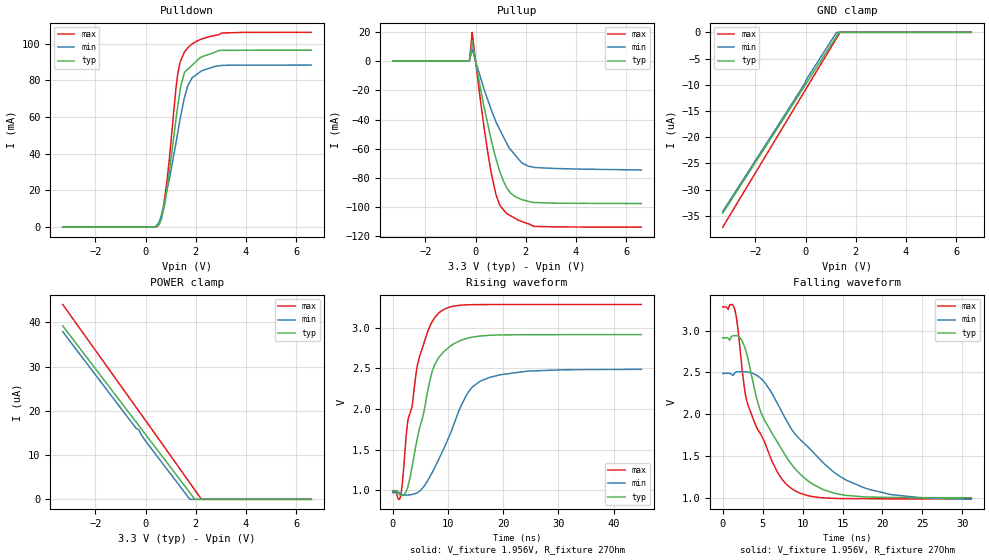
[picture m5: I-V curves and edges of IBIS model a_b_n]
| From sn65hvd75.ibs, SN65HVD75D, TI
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[Model]   a_b_n
Model_type   I/O
Polarity   Non-Inverting
Enable   Active-High
Vinl = 0.8
Vinh = 2.0
Vmeas = 1.65
Vref = 1.65
Cref = 50pF
Rref = 27
|   typ   min   max
|   (nom PVT)   (fast PVT)   (slow PVT)
C_comp   2.134e-11   2.058e-11   2.134e-11
|ON state : BUFFER OUTPUT TURNED HIGH
|C_comp   2.134e-11   2.058e-11   2.134e-11
|OFF state: BUFFER IN HIGH IMPEDANCE
|C_comp   1.142e-11   1.069e-11   1.206e-11
| Where nom  PVT is Nominal Process, 3.3V, 27C
|   Fast PVT is Strong Process,  3.6V, -40C
|   Slow PVT is Weak Process,   3V, 125C
[Voltage Range]   3.3   3   3.6
|Ambient Temperature   25   125   -40
|Junction Temperature
[Temperature Range]   27   125   -40
[Pullup Reference]   3.3   3   3.6
[Pulldown Reference]   0   0   0
[Power Clamp Reference]   3.3   3   3.6
[GND Clamp Reference]   0   0   0
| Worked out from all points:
|   slope of the pulldown table from 0 to 0.495 V, typ, clamps not added: 482 ohm
|   slope of the pullup table from 0 to 0.495 V, typ, clamps not added: 11.3 ohm
|   falling waveform, V_fixture 1.956V, R_fixture 27Ohm: 20-80 % time 5.29ns typ, 7.74ns min, 4.01ns max; typ from 2.92 V to 0.998 V
|   rising waveform, V_fixture 1.956V, R_fixture 27Ohm: 20-80 % time 3.78ns typ, 5.92ns min, 3.54ns max; typ from 0.997 V to 2.91 V
[Pulldown]
|   Voltage   I(typ)   I(min)   I(max)
-3.3V     0A         0A         0A
478.8mV   881.8uA    1.608mA    490.4uA
633.6mV   4.473mA    6.787mA    5.518mA
849.6mV   20.36mA    20.02mA    24.85mA
1.202V    57.94mA    45.29mA    74.75mA
1.285V    66.34mA    51.87mA    83.81mA
1.399V    76.97mA    60.61mA    90.81mA
1.554V    84.49mA    70.97mA    95.7mA
1.854V    88.36mA    81.44mA    99.95mA
2.168V    92.42mA    84.62mA    102.3mA
2.934V    96.41mA    88.05mA    105.1mA
6.6V      96.53mA    88.41mA    106.3mA
[GND Clamp]
|   Voltage   I(typ)   I(min)   I(max)
-3.3V     -34.49uA   -34.15uA   -37.14uA
-162mV    -11.16uA   -10.73uA   -12.21uA
111mV     -9.118uA   -8.406uA   -10.04uA
1.236V    -746.4nA   -6.684nA   -1.095uA
1.333V    -22.23nA   0A         -321.6nA
1.372V    0A         0A         -15.83nA
6.6V      0A         0A         0A
[Pullup]
|   Voltage   I(typ)   I(min)   I(max)
-3.3V     0A         0A         0A
-248.4mV  0A         0A         0A
-133.2mV  13.34mA    8.273mA    19.82mA
64.8mV    -6.244mA   -3.735mA   -9.275mA
342mV     -31.73mA   -19.41mA   -45.91mA
633.6mV   -54.97mA   -33.82mA   -77.49mA
802.8mV   -66.31mA   -41.19mA   -90.85mA
939.6mV   -74.34mA   -46.13mA   -97.84mA
1.213V    -85.9mA    -55.41mA   -104.1mA
1.554V    -92.65mA   -63.94mA   -107.6mA
2.115V    -96.23mA   -72.14mA   -111.7mA
6.6V      -97.64mA   -74.6mA    -113.8mA
[POWER Clamp]
|   Voltage   I(typ)   I(min)   I(max)
-3.3V     39.2uA     37.89uA    44.02uA
-378mV    17.47uA    16.05uA    20.8uA
-264mV    16.62uA    15.69uA    19.89uA
-150mV    15.78uA    14.44uA    18.99uA
6mV       14.61uA    13.14uA    17.75uA
1.761V    1.513uA    15.72nA    3.718uA
1.964V    2.365nA    0A         2.098uA
2.225V    0A         0A         12.85nA
6.6V      0A         0A         0A
[Ramp]
R_load = 27
|   typ   min   max
dV/dt_r   1.32254/4.33263e-09   0.977856/7.13635e-09   1.58731/3.88744e-09
dV/dt_f   1.15015/5.29718e-09   0.908154/7.76592e-09   1.38004/4.01751e-09
[Falling Waveform]
V_fixture = 1.956V
V_fixture_min = 1.731V
V_fixture_max = 2.134V
R_fixture = 27Ohm
C_fixture = 0F
|   Time   V(typ)   V(min)   V(max)
0s        2.915V     2.488V     3.285V
1.5ns     2.94V      2.492V     3.258V
2.44ns    2.876V     2.509V     2.531V
3.05ns    2.707V     2.506V     2.148V
4.79ns    2.02V      2.427V     1.753V
6.95ns    1.65V      2.11V      1.288V
8.58ns    1.402V     1.823V     1.11V
12.39ns   1.104V     1.435V     997.9mV
17.6ns    1.009V     1.121V     986mV
31.12ns   998.1mV    978.9mV    984.8mV
[Rising Waveform]
V_fixture = 1.956V
V_fixture_min = 1.731V
V_fixture_max = 2.134V
R_fixture = 27Ohm
C_fixture = 0F
|   Time   V(typ)   V(min)   V(max)
0s        996.9mV    973.6mV    983.5mV
1.4ns     941.1mV    969.6mV    922.1mV
1.73ns    939.6mV    951.3mV    1.079V
2.47ns    992.3mV    943.4mV    1.699V
4.91ns    1.777V     994mV      2.653V
7.12ns    2.454V     1.218V     3.07V
8.62ns    2.655V     1.424V     3.195V
13.18ns   2.863V     2.151V     3.279V
15.85ns   2.897V     2.343V     3.283V
45ns      2.914V     2.487V     3.284V
